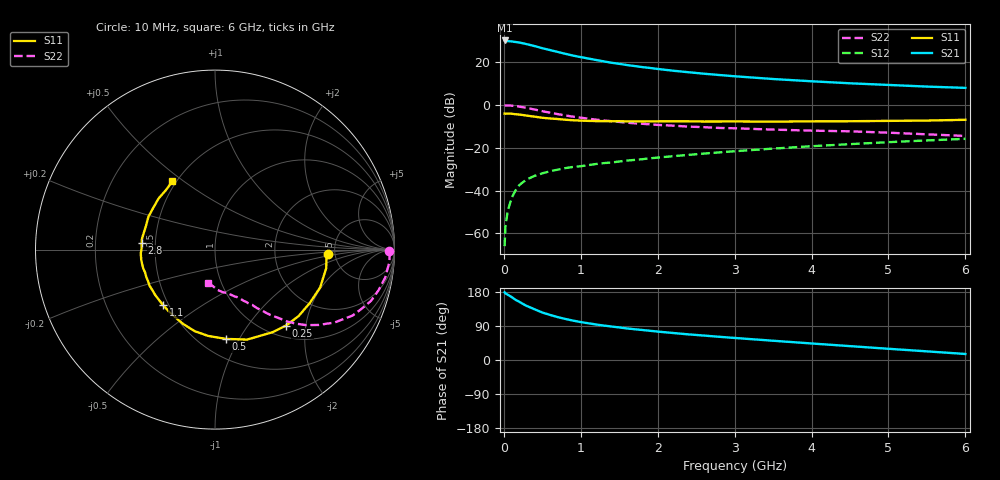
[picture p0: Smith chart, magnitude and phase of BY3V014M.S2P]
! SIEMENS Small Signal Semiconductors
! BFY420
! Si NPN RF SIEGET Grounded Emitter Transistor in MICRO-X
! VCE = 3 V  IC = 14 mA
! Common Emitter S-Parameters:  October  1996
# GHz  S  MA  R  50
!  f  S11  S21  S12  S22
! GHz  MAG  ANG  MAG  ANG  MAG  ANG  MAG  ANG
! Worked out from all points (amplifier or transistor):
!   36 points, 10 MHz to 6 GHz, reference 50 ohm
!   highest |S21| = 30.1 dB at 10 MHz (marker M1)
!   |S21| within 3 dB of that: start of sweep to 437.6 MHz
!   unconditionally stable (mu >= 1): start of sweep to 10.96 MHz; 2.28 GHz to end of sweep
!   at 250 MHz: K = 0.25, MSG = 32.4 dB, |S12| = -36.1 dB
!   at 1.4 GHz: K = 0.84, MSG = 23.3 dB, |S12| = -26.9 dB
!   at 6 GHz: K = 1.08, MAG = 10.2 dB, |S12| = -15.8 dB
!   S11 on the Smith chart (normalised r, x): 10 MHz: 4.34, -0.31; 250 MHz: 1.22, -1.56; 500 MHz: 0.66, -0.88; 1.1 GHz: 0.47, -0.35; 2.8 GHz: 0.42, +0.04; 6 GHz: 0.48, +0.45
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0.01  0.6272 -2.0  32.11 178.7  0.0005 84.1  0.971 -0.6
0.02  0.6226 -4.1  31.73 176.1  0.0014 73.5  0.9746 -1.6
0.1  0.6228 -19.7  30.54 166.3  0.0066 80.8  0.9608 -9.4
0.15  0.6063 -29.4  29.59 159.1  0.0099 75.2  0.9387 -14.0
0.2  0.5951 -38.5  28.73 153.8  0.0133 73.8  0.9149 -18.2
0.25  0.5796 -46.9  27.52 147.7  0.0157 68.7  0.8798 -22.1
0.3  0.5611 -55.1  26.25 142.5  0.0182 68.3  0.8503 -25.6
0.4  0.5323 -70.4  23.73 133.8  0.022 62.7  0.7799 -31.4
0.5  0.5011 -83.1  21.16 125.3  0.0252 59.8  0.7142 -36.0
0.6  0.4825 -94.5  19.14 119.0  0.0282 57.3  0.6588 -39.7
0.7  0.4685 -103.9  17.32 113.2  0.0307 55.8  0.6105 -42.5
0.8  0.4507 -113.2  15.62 108.3  0.0334 54.5  0.5674 -44.9
0.9  0.438 -120.0  14.22 103.9  0.0356 53.9  0.5318 -46.5
1.1  0.4235 -133.2  12.13 96.8  0.0393 54.2  0.4758 -49.8
1.3  0.4186 -142.6  10.41 90.9  0.0437 53.7  0.4329 -52.1
1.6  0.4123 -154.7  8.554 83.3  0.0501 53.7  0.3847 -55.3
2.2  0.4149 -172.1  6.302 71.3  0.0634 53.1  0.3277 -60.7
2.8  0.41 174.7  5.001 61.3  0.0777 51.0  0.2896 -65.5
3.5  0.4065 161.9  4.031 50.8  0.0953 47.3  0.2651 -70.9
4.5  0.4154 145.9  3.201 36.6  0.1212 40.5  0.2416 -79.6
5.5  0.4308 128.9  2.682 22.8  0.148 32.1  0.2057 -92.6
6  0.4491 121.9  2.503 15.9  0.1613 27.7  0.1883 -101.3
